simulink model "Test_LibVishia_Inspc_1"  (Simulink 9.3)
settings: Solver=FixedStepDiscrete  StartTime=0.0  StopTime=0.5  FixedStep=Tstep  RelTol=1e-3  EnableMultiTasking=on
InitFcn:
  | Test_LibVishia_Inspc.Test_LibVishia_Inspc_init();
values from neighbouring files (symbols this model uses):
  Tstep = 0.000050    (= 5e-05)    [Test_LibVishia_Inspc_init.m]    (also in Test_SharedMemVS_init.m; InspcCtrl_init.m = 0.0001; TestOrthOscObjO_init.m = 0.0005; stimuli_Smlk.m = 0.001)
libraries: libVishia_Inspc x3

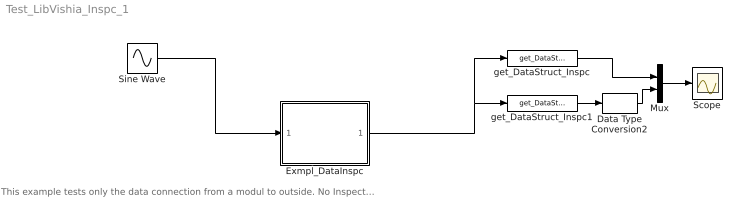
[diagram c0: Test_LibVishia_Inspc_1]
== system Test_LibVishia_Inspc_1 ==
  note: This example tests only the data connection from a modul to outside. No Inspector access itself. Test it independently.
  Data Type Conversion2 : DataTypeConversion  OutDataTypeStr=single
  Exmpl_DataInspc : Subsystem
  Mux : Mux  Inputs=2
  Scope : Scope
  Sine Wave : Sin  Frequency=50*2*pi  SampleTime=Tstep
  get_DataStruct_Inspc : libVishia_Inspc/get_DataStruct_Inspc  show='name'  Tstep=Tstep  name1='name :F'  headerfile=''
  get_DataStruct_Inspc1 : libVishia_Inspc/get_DataStruct_Inspc  show='name2'  Tstep=Tstep  name1='name2 : I'  headerfile=''
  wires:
  get_DataStruct_Inspc/1 -> Mux/1
  Mux/1 -> Scope/1
  get_DataStruct_Inspc1/1 -> Data Type Conversion2/1
  Data Type Conversion2/1 -> Mux/2
  Exmpl_DataInspc/1(Out1) -> get_DataStruct_Inspc/1, get_DataStruct_Inspc1/1
  Sine Wave/1 -> Exmpl_DataInspc/1(In1)

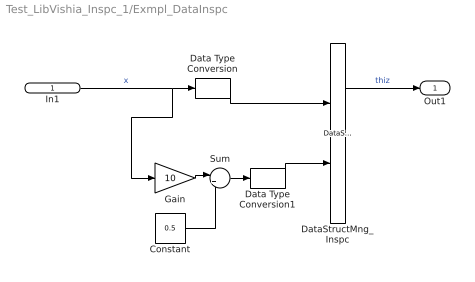
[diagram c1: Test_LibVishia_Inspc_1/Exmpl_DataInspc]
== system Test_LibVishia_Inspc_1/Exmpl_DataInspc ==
  In1 : Inport  OutDataTypeStr=double
  Constant : Constant  Value=0.5
  Data Type Conversion : DataTypeConversion  OutDataTypeStr=single
  Data Type Conversion1 : DataTypeConversion  OutDataTypeStr=int32
  DataStructMng_Inspc : libVishia_Inspc/DataStructMng_Inspc  dirGenSource=dstPathGenDataStruct  typeData='TypeData'  inherit=off  chain=off  inputs=|
      | name:F;           //simple variable, type from connection 
      | name2 :I;
  Gain : Gain  Gain=10
  Sum : Sum  Inputs=|++
  Out1 : Outport  OutDataTypeStr=uint32
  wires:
  Sum/1 -> Data Type Conversion1/1
  Data Type Conversion/1 -> DataStructMng_Inspc/1
  In1/1 -> Gain/1, Data Type Conversion/1  "x"
  DataStructMng_Inspc/1 -> Out1/1  "thiz"
  Constant/1 -> Sum/2
  Data Type Conversion1/1 -> DataStructMng_Inspc/2
  Gain/1 -> Sum/1
